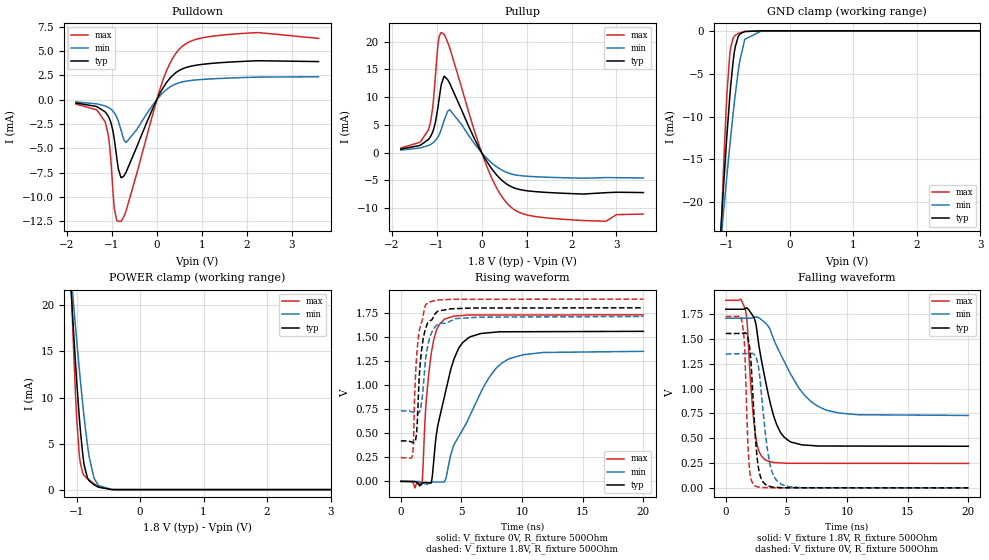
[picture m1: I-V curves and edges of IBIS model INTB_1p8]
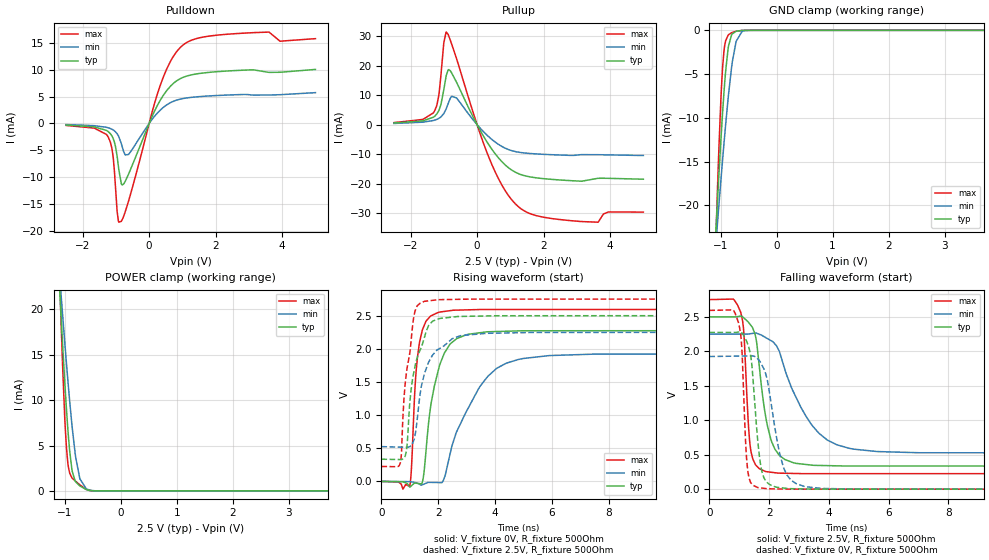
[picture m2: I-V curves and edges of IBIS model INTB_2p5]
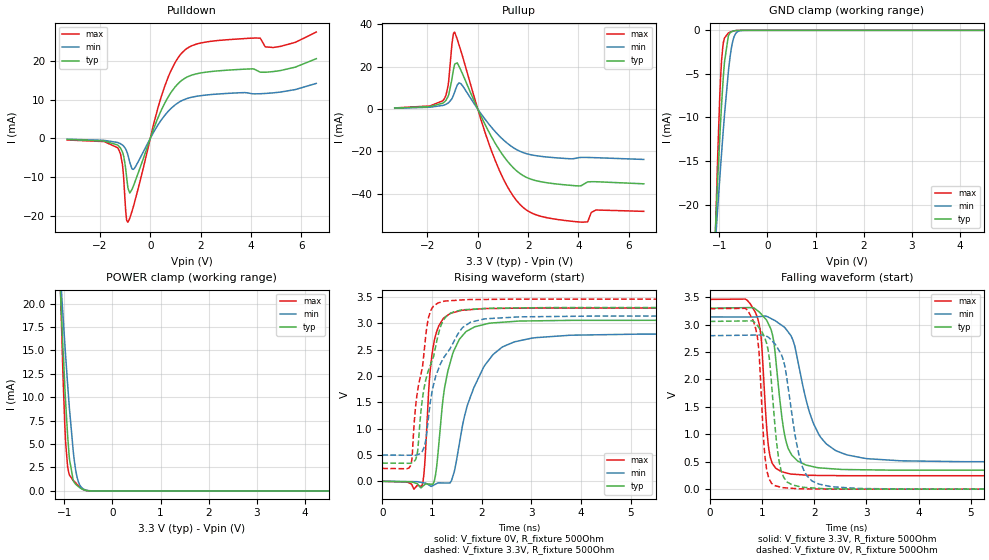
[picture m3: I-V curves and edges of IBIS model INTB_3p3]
|Texas Instruments Incorporated
| Marketing part#   Digital Voltage Range   Package-type   #pins
| LDC1101   1.71V - 3.46V   WSON   10
[IBIS Ver]   4.1
[File name]   ldc1101.ibs
[File Rev]   1.0
[Date]   10/21/2014
[Source]
| Texas Instruments Incorporated.
| 12500 TI Blvd
| Dallas, TX -75243
[Notes]   Revision History:
| Rev 1.0: 10/21/2014
| - Initial version of the model
| - Model generated from simulations in TISPICE
| - C_comp although listed in numerical order of value are
|   obtained from varying PVT conditions. For PVT conditions for
|   each specific value refer the buffer description under
|   respective [Model]. IBIS model user is responsible for using
|   appropriate C_comp to simulate for Signal Integrity.
| - Warnings regarding combined Non-monotonicity of various models have been
|   reviewd and considered minor and can be ignored.
| - Model names with a trailing _1p8 contains the model for
|   1.8V operation. Model names with a trailing _2p5 contains the model
|   for 2.5V operation.Model names with a trailing _3p3 contains the model
|   for 3.3V operation.
[Disclaimer]
| This model is designed as an aid for customers of Texas Instruments.
| TI and its licensors and suppliers make no warranties, either expressed
| or implied, with respect to this  model, including the warranties of
| merchantability or fitness for a particular purpose. The model is
| provided solely on an "as is" basis. The entire risk as to its quality
| and performance is with the customer.
[Copyright]
 (C) Copyright 2014 Texas Instruments Incorporated.All rights reserved.
|   Device
[Component] LDC1101
[Manufacturer]   TI
[Package]  |QFN   64
|   typ   min   max
R_pkg   0.067   0.027   0.083
L_pkg   0.937nH   0.593nH   1.143nH
C_pkg   0.144pF   0.126pF   0.200pF
[Pin]  signal_name   model_name   R_pin   L_pin   C_pin
1   SDO/INTB   INTB   0.07225   0.9423nF   0.10569pF
2   CLKIN   INPUT   0.06963   0.90122nF   0.11966pF
3   SCLK   INPUT   0.06783   0.8751nF   0.1181pF
4   SDI   INPUT   0.06766   0.87334nF   0.11843pF
5   CSB   INPUT   0.07162   0.93329nF   0.10577pF
6   INB   NC   0.03667   0.6676nF   0.1339pF
7   INA   NC   0.03767   0.69067nF   0.16038pF
8   GND   GND   0.03452   0.60581nF   0.15824pF
9   VDD   POWER   0.0342   0.59712nF   0.15278pF
10   CLDO   NC   0.0717   0.92726nF   0.10658pF
|   Model Selectors
[Model Selector]  INTB
INTB_1p8  output buffer at 1.8V operation.
INTB_2p5  output buffer at 2.5V operation.
INTB_3p3  output buffer at 3.3V operation.
[Model Selector]  INPUT
SCLK_1p8  output buffer at 1.8V operation.
SCLK_2p5  output buffer at 2.5V operation.
SCLK_3p3  output buffer at 3.3V operation.
| Models and submodels in the file (6): INTB_1p8 (I/O), INTB_2p5 (I/O), INTB_3p3 (I/O), SCLK_1p8 (Input), SCLK_2p5 (Input), SCLK_3p3 (Input)
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|   Model
[Model]   INTB_1p8
Model_type   I/O
Polarity   Non-Inverting
Enable   Active-Low
Vinl = 0.54
Vinh = 1.26
Vmeas = 0.9
Vref = 0
Cref = 1pF
Rref = 100000
|   typ   min   max
C_comp   0.827pF   0.793pF   0.868pF
[Voltage Range]   1.8   1.71   1.89
[Temperature Range]   27   125   -40
[Pullup Reference]   1.8   1.71   1.89
[Pulldown Reference]   0   0   0
[Power Clamp Reference]   1.8   1.71   1.89
[GND Clamp Reference]   0   0   0
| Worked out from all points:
|   slope of the pulldown table from 0 to 0.27 V, typ, clamps not added: 130 ohm
|   slope of the pullup table from 0 to 0.27 V, typ, clamps not added: 80 ohm
|   GND clamp passes 1 mA (typ) near -0.83 V on its own axis
|   POWER clamp passes 1 mA (typ) near -0.80 V on its own axis
|   falling waveform, V_fixture 1.8V, R_fixture 500Ohm: 20-80 % time 1.4ns typ, 2.66ns min, 587ps max; typ from 1.8 V to 0.419 V
|   rising waveform, V_fixture 0V, R_fixture 500Ohm: 20-80 % time 1.54ns typ, 3.19ns min, 692ps max; typ from 0 V to 1.56 V
|   rising waveform, V_fixture 1.8V, R_fixture 500Ohm: 20-80 % time 531ps typ, 637ps min, 447ps max; typ from 0.419 V to 1.8 V
|   falling waveform, V_fixture 0V, R_fixture 500Ohm: 20-80 % time 493ps typ, 755ps min, 297ps max; typ from 1.56 V to 0 V
[Pulldown]
|   Voltage   I(typ)   I(min)   I(max)
-1.8V     -336.3uA   -230.4uA   -447.7uA
-1.357V   -678.6uA   -412.5uA   -1.012mA
-1.152V   -1.24mA    -641.7uA   -2.261mA
-1.049V   -2.004mA   -876.5uA   -4.803mA
-946.8mV  -4.023mA   -1.336mA   -11.16mA
-892.8mV  -5.91mA    -1.773mA   -12.37mA
-801mV    -7.966mA   -3.049mA   -12.48mA
-682.2mV  -7.425mA   -4.392mA   -11.39mA
117mV     1.045mA    623.4uA    1.749mA
538.2mV   3.104mA    1.8mA      5.371mA
1.899V    3.933mA    2.274mA    6.804mA
3.6V      3.919mA    2.358mA    6.302mA
[GND Clamp]
|   Voltage   I(typ)   I(min)   I(max)
-1.8V     -120.6mA   -88.57mA   -196.3mA
-1.093V   -24.03mA   -25.16mA   -25.67mA
-1.055V   -19.45mA   -22.03mA   -18.1mA
-995.4mV  -12.68mA   -17.26mA   -8.035mA
-946.8mV  -7.79mA    -13.52mA   -2.868mA
-930.6mV  -6.358mA   -12.32mA   -1.935mA
-876.6mV  -2.636mA   -8.545mA   -652.2uA
-811.8mV  -641.6uA   -4.675mA   -304.6uA
-784.8mV  -359uA     -3.37mA    -230.3uA
-709.2mV  -81.9uA    -992uA     -81.84uA
-444.6mV  -100.8nA   -2.623uA   -20.3nA
3.6V      0A         0A         0A
[Pullup]
|   Voltage   I(typ)   I(min)   I(max)
-1.8V     652.3uA    478.7uA    841.9uA
-1.384V   1.299mA    843.4uA    1.858mA
-1.184V   2.391mA    1.309mA    4.139mA
-1.093V   3.712mA    1.732mA    8.059mA
-973.8mV  8.197mA    2.83mA     19.49mA
-898.2mV  12.34mA    4.232mA    21.64mA
-833.4mV  13.78mA    5.911mA    21.28mA
-709.2mV  12.44mA    7.72mA     18.83mA
68.4mV    -966.5uA   -617uA     -1.527mA
613.8mV   -5.931mA   -3.713mA   -9.529mA
1.975V    -7.359mA   -4.541mA   -12.08mA
3.6V      -7.18mA    -4.556mA   -11.05mA
[POWER Clamp]
|   Voltage   I(typ)   I(min)   I(max)
-1.8V     116.8mA    87.13mA    188mA
-1.093V   22.48mA    23.87mA    23.88mA
-1.06V    18.67mA    21.21mA    17.71mA
-1.001V   12.14mA    16.47mA    8.209mA
-946.8mV  7.028mA    12.4mA     3.206mA
-903.6mV  3.914mA    9.363mA    1.825mA
-876.6mV  2.568mA    7.609mA    1.493mA
-801mV    957uA      3.559mA    1.042mA
-725.4mV  531.3uA    1.252mA    646.1uA
-655.2mV  264.8uA    440.2uA    306.4uA
-444.6mV  3.686uA    12.87uA    1.63uA
3.6V      0A         0A         0A
[Ramp]
R_load = 500
|   typ   min   max
dV/dt_r   0.933471/1.5386e-09   0.809123/3.18535e-09   1.03613/6.85503e-10
dV/dt_f   0.828579/1.39636e-09   0.588178/2.65405e-09   0.9861/5.85084e-10
[Falling Waveform]
V_fixture = 1.8V
V_fixture_min = 1.71V
V_fixture_max = 1.89V
R_fixture = 500Ohm
C_fixture = 0F
|   Time   V(typ)   V(min)   V(max)
0s        1.8V       1.71V      1.89V
1.219ns   1.799V     1.71V      1.902V
1.63ns    1.808V     1.71V      1.788V
2.415ns   1.686V     1.72V      562.5mV
3.241ns   1.099V     1.664V     283.3mV
3.994ns   708.3mV    1.484V     255.4mV
4.823ns   509.5mV    1.273V     249.3mV
6.519ns   431.2mV    930.5mV    247.5mV
8.115ns   421.7mV    792mV      247.4mV
20ns      419mV      729.7mV    246.5mV
[Rising Waveform]
V_fixture = 0V
V_fixture_min = 0V
V_fixture_max = 0V
R_fixture = 500Ohm
C_fixture = 0F
|   Time   V(typ)   V(min)   V(max)
0s        3.042nV    52.01nV    1.465nV
1.72ns    -21.89mV   -11.15mV   -32.73mV
2.079ns   -12.56mV   -28.1mV    808.2mV
2.481ns   -16.96mV   -12.94mV   1.302V
2.927ns   483.4mV    -6.927mV   1.564V
3.566ns   863.7mV    -7.019mV   1.678V
4.336ns   1.249V     367.4mV    1.713V
5.108ns   1.44V      539mV      1.721V
8.246ns   1.551V     1.219V     1.725V
20ns      1.556V     1.349V     1.727V
[Rising Waveform]
V_fixture = 1.8V
V_fixture_min = 1.71V
V_fixture_max = 1.89V
R_fixture = 500Ohm
C_fixture = 0F
|   Time   V(typ)   V(min)   V(max)
0s        419mV      729.7mV    246.5mV
959.8ps   405.7mV    717.9mV    272.1mV
1.041ns   402.7mV    714.2mV    410.8mV
1.213ns   426.2mV    706.5mV    1.108V
1.395ns   723.9mV    702.1mV    1.436V
1.685ns   1.338V     797.6mV    1.639V
2.207ns   1.643V     1.399V     1.854V
2.906ns   1.749V     1.615V     1.879V
4.522ns   1.791V     1.688V     1.889V
20ns      1.8V       1.71V      1.89V
[Falling Waveform]
|Gnd
V_fixture = 0V
V_fixture_min = 0V
V_fixture_max = 0V
R_fixture = 500Ohm
C_fixture = 0F
|   Time   V(typ)   V(min)   V(max)
0s        1.556V     1.349V     1.727V
1.354ns   1.557V     1.352V     1.663V
1.56ns    1.562V     1.353V     1.409V
1.795ns   1.524V     1.353V     546mV
1.927ns   1.446V     1.354V     229.4mV
2.415ns   563.4mV    1.332V     19.53mV
2.764ns   154.3mV    1.161V     6.042mV
3.607ns   15.45mV    260.5mV    487.1uV
4.559ns   2.439mV    37.84mV    407.4uV
20ns      13.76nV    93.77nV    4.829nV
|   Model
[Model]   INTB_2p5
Model_type   I/O
Polarity   Non-Inverting
Enable   Active-Low
Vinl = 0.75
Vinh = 1.75
Vmeas = 1.25
Vref = 0
Cref = 1pF
Rref = 100000
|   typ   min   max
C_comp   0.827pF   0.793pF   0.868pF
[Voltage Range]   2.5   2.25   2.75
[Temperature Range]   27   125   -40
[Pullup Reference]   2.5   2.25   2.75
[Pulldown Reference]   0   0   -0
[Power Clamp Reference]   2.5   2.25   2.75
[GND Clamp Reference]   0   0   0
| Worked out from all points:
|   slope of the pulldown table from 0 to 0.375 V, typ, clamps not added: 79 ohm
|   slope of the pullup table from 0 to 0.375 V, typ, clamps not added: 52.1 ohm
|   GND clamp passes 1 mA (typ) near -0.82 V on its own axis
|   POWER clamp passes 1 mA (typ) near -0.81 V on its own axis
|   falling waveform, V_fixture 2.5V, R_fixture 500Ohm: 20-80 % time 432ps typ, 1.14ns min, 184ps max; typ from 2.5 V to 0.334 V
|   rising waveform, V_fixture 0V, R_fixture 500Ohm: 20-80 % time 539ps typ, 1.26ns min, 242ps max; typ from 0 V to 2.27 V
|   rising waveform, V_fixture 2.5V, R_fixture 500Ohm: 20-80 % time 503ps typ, 561ps min, 339ps max; typ from 0.334 V to 2.5 V
|   falling waveform, V_fixture 0V, R_fixture 500Ohm: 20-80 % time 263ps typ, 478ps min, 153ps max; typ from 2.27 V to 0 V
[Pulldown]
|   Voltage   I(typ)   I(min)   I(max)
-2.5V     -286uA     -200.7uA   -364.7uA
-1.653V   -630.8uA   -404.1uA   -862uA
-1.225V   -1.546mA   -811.9uA   -2.588mA
-1.09V    -2.686mA   -1.17mA    -5.892mA
-962.5mV  -6.113mA   -1.915mA   -16.44mA
-910mV    -8.699mA   -2.493mA   -18.41mA
-812.5mV  -11.47mA   -4.284mA   -17.99mA
-617.5mV  -9.426mA   -5.786mA   -14.45mA
327.5mV   4.261mA    2.451mA    6.995mA
957.5mV   8.425mA    4.574mA    14.31mA
2.728V    9.913mA    5.387mA    16.81mA
5V        10.08mA    5.752mA    15.83mA
[GND Clamp]
|   Voltage   I(typ)   I(min)   I(max)
-2.5V     -220.6mA   -154mA     -373.8mA
-1.143V   -30.31mA   -29.38mA   -36.4mA
-1.067V   -20.97mA   -23.08mA   -20.57mA
-1.052V   -19.17mA   -21.85mA   -17.66mA
-992.5mV  -12.37mA   -17.03mA   -7.632mA
-962.5mV  -9.283mA   -14.71mA   -4.145mA
-940mV    -7.174mA   -13.01mA   -2.432mA
-865mV    -2.088mA   -7.79mA    -553uA
-805mV    -551.9uA   -4.326mA   -284.3uA
-722.5mV  -106.5uA   -1.271mA   -101.6uA
-550mV    -2.125uA   -30.09uA   -1.294uA
5V        0A         0A         0A
[Pullup]
|   Voltage   I(typ)   I(min)   I(max)
-2.5V     535.2uA    389.6uA    684.5uA
-1.285V   2.751mA    1.489mA    4.495mA
-1.15V    4.763mA    2.122mA    9.98mA
-1V       11.85mA    3.753mA    27.79mA
-925mV    16.73mA    5.437mA    31.41mA
-850mV    18.68mA    7.715mA    30.06mA
-617.5mV  14.39mA    9.063mA    22.43mA
327.5mV   -6.394mA   -3.871mA   -10.33mA
1.167V    -16.24mA   -9.188mA   -27.08mA
1.798V    -18.08mA   -9.952mA   -30.93mA
3.147V    -19.2mA    -10.19mA   -32.9mA
5V        -18.52mA   -10.48mA   -29.68mA
[POWER Clamp]
|   Voltage   I(typ)   I(min)   I(max)
-2.5V     214.8mA    152.6mA    359mA
-1.15V    29.5mA     28.69mA    35.7mA
-1.075V   20.4mA     22.42mA    20.47mA
-1.067V   19.52mA    21.81mA    19.06mA
-1V       12.05mA    16.41mA    8.104mA
-970mV    9.092mA    14.12mA    4.83mA
-940mV    6.469mA    11.9mA     2.87mA
-872.5mV  2.406mA    7.354mA    1.458mA
-805mV    992.7uA    3.733mA    1.062mA
-730mV    551.7uA    1.342mA    671.2uA
-617.5mV  161.2uA    254.8uA    175.1uA
5V        0A         0A         0A
[Ramp]
R_load = 500
|   typ   min   max
dV/dt_r   1.36448/5.34294e-10   1.15475/1.25777e-09   1.55607/2.4163e-10
dV/dt_f   1.29952/4.27066e-10   1.0354/1.13003e-09   1.51514/1.83827e-10
[Falling Waveform]
V_fixture = 2.5V
V_fixture_min = 2.25V
V_fixture_max = 2.75V
R_fixture = 500Ohm
C_fixture = 0F
|   Time   V(typ)   V(min)   V(max)
0s        2.5V       2.25V      2.75V
1.042ns   2.512V     2.249V     2.574V
1.158ns   2.483V     2.249V     2.244V
1.385ns   2.379V     2.256V     567.8mV
1.583ns   2.128V     2.262V     336.1mV
1.862ns   1.11V      2.205V     259.5mV
2.521ns   431.3mV    1.743V     230.8mV
3.459ns   347.2mV    913.6mV    225.4mV
4.681ns   335.5mV    592.7mV    225.4mV
20ns      334.1mV    524.3mV    224.8mV
[Rising Waveform]
V_fixture = 0V
V_fixture_min = 0V
V_fixture_max = 0V
R_fixture = 500Ohm
C_fixture = 0F
|   Time   V(typ)   V(min)   V(max)
0s        2.164nV    45.82nV    1.193nV
995.4ps   -84.78mV   -3.588mV   -62.6mV
1.202ns   -26.46mV   -18.48mV   1.549V
1.334ns   -33.31mV   -42.21mV   2.076V
1.473ns   52.44mV    -45.51mV   2.317V
1.741ns   1.154V     -14.99mV   2.496V
1.988ns   1.65V      -17.49mV   2.547V
3.459ns   2.241V     1.423V     2.592V
4.833ns   2.27V      1.84V      2.592V
20ns      2.274V     1.925V     2.593V
[Rising Waveform]
V_fixture = 2.5V
V_fixture_min = 2.25V
V_fixture_max = 2.75V
R_fixture = 500Ohm
C_fixture = 0F
|   Time   V(typ)   V(min)   V(max)
0s        334.1mV    524.3mV    224.8mV
663.6ps   329.5mV    516.6mV    275.6mV
876.9ps   451.6mV    514.1mV    1.626V
1.004ns   1.212V     524.2mV    1.954V
1.13ns    1.623V     609.1mV    2.459V
1.507ns   2.162V     1.611V     2.715V
1.807ns   2.419V     1.907V     2.731V
2.492ns   2.478V     2.152V     2.744V
3.705ns   2.495V     2.233V     2.749V
20ns      2.5V       2.25V      2.75V
[Falling Waveform]
|Gnd
V_fixture = 0V
V_fixture_min = 0V
V_fixture_max = 0V
R_fixture = 500Ohm
C_fixture = 0F
|   Time   V(typ)   V(min)   V(max)
0s        2.274V     1.925V     2.593V
972.3ps   2.28V      1.93V      2.417V
1.087ns   2.268V     1.931V     2.039V
1.276ns   2.113V     1.932V     298.4mV
1.417ns   1.822V     1.933V     78.44mV
1.607ns   763.7mV    1.897V     25.95mV
1.819ns   171.4mV    1.75V      12.86mV
2.492ns   15.68mV    303.6mV    1.677mV
3.165ns   3.772mV    41.04mV    385.7uV
20ns      6.394nV    60.83nV    2.527nV
|   Model
[Model]   INTB_3p3
Model_type   I/O
Polarity   Non-Inverting
Enable   Active-Low
Vinl = 0.99
Vinh = 2.31
Vmeas = 1.65
Vref = 0
Cref = 1pF
Rref = 100000
|   typ   min   max
C_comp   0.827pF   0.793pF   0.868pF
[Voltage Range]   3.3   3.14   3.46
[Temperature Range]   27   125   -40
[Pullup Reference]   3.3   3.14   3.46
[Pulldown Reference]   0   0   0
[Power Clamp Reference]   3.3   3.14   3.46
[GND Clamp Reference]   0   0   0
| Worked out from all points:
|   slope of the pulldown table from 0 to 0.495 V, typ, clamps not added: 61.8 ohm
|   slope of the pullup table from 0 to 0.495 V, typ, clamps not added: 41.4 ohm
|   GND clamp passes 1 mA (typ) near -0.82 V on its own axis
|   POWER clamp passes 1 mA (typ) near -0.81 V on its own axis
|   falling waveform, V_fixture 3.3V, R_fixture 500Ohm: 20-80 % time 223ps typ, 447ps min, 136ps max; typ from 3.3 V to 0.346 V
|   rising waveform, V_fixture 0V, R_fixture 500Ohm: 20-80 % time 297ps typ, 569ps min, 164ps max; typ from 0 V to 3.06 V
|   rising waveform, V_fixture 3.3V, R_fixture 500Ohm: 20-80 % time 364ps typ, 509ps min, 254ps max; typ from 0.346 V to 3.3 V
|   falling waveform, V_fixture 0V, R_fixture 500Ohm: 20-80 % time 181ps typ, 289ps min, 122ps max; typ from 3.06 V to 0 V
[Pulldown]
|   Voltage   I(typ)   I(min)   I(max)
-3.3V     -247.8uA   -199.8uA   -395.2uA
-1.29V    -1.724mA   -1.053mA   -2.459mA
-1.102V   -3.533mA   -1.699mA   -6.822mA
-973.5mV  -7.984mA   -2.771mA   -18.83mA
-894.3mV  -12.38mA   -4.103mA   -21.53mA
-815.1mV  -14.05mA   -6.096mA   -20.54mA
-636.9mV  -11.66mA   -7.736mA   -16.72mA
432.3mV   7.171mA    4.689mA    10.63mA
1.264V    14.98mA    9.747mA    22.03mA
3.897V    17.85mA    11.68mA    25.74mA
5.174V    17.45mA    11.92mA    23.66mA
6.6V      20.5mA     14.15mA    27.34mA
[GND Clamp]
|   Voltage   I(typ)   I(min)   I(max)
-3.3V     -336.1mA   -229.7mA   -578mA
-1.082V   -22.78mA   -24.31mA   -23.57mA
-1.073V   -21.57mA   -23.49mA   -21.57mA
-1.043V   -18.03mA   -21.05mA   -15.85mA
-993.3mV  -12.45mA   -17.09mA   -7.742mA
-953.7mV  -8.434mA   -14.04mA   -3.382mA
-894.3mV  -3.652mA   -9.739mA   -877.6uA
-815.1mV  -690.8uA   -4.848mA   -315.1uA
-765.6mV  -244.4uA   -2.582mA   -184.9uA
-676.5mV  -41.86uA   -513.7uA   -44.42uA
-518.1mV  -896.7nA   -14.44uA   -415.7nA
6.6V      0A         0A         0A
[Pullup]
|   Voltage   I(typ)   I(min)   I(max)
-3.3V     449.8uA    359.3uA    530.3uA
-1.36V    3.018mA    1.808mA    4.322mA
-1.181V   5.896mA    2.797mA    10.87mA
-1.023V   14.5mA     4.996mA    30.9mA
-924mV    20.8mA     7.827mA    36.28mA
-676.5mV  18.44mA    12.01mA    27.64mA
570.9mV   -13.6mA    -8.959mA   -20.48mA
1.68V     -30.4mA    -19.91mA   -44.99mA
2.472V    -34.16mA   -22.23mA   -50.43mA
4.155V    -35.82mA   -22.8mA    -53.33mA
4.699V    -34.25mA   -22.93mA   -47.57mA
6.6V      -35.24mA   -23.75mA   -48.22mA
[POWER Clamp]
|   Voltage   I(typ)   I(min)   I(max)
-3.3V     327.9mA    228.3mA    556.1mA
-1.082V   21.27mA    23.03mA    21.89mA
-1.073V   20.1mA     22.21mA    20mA
-1.033V   15.58mA    19.01mA    12.97mA
-993.3mV  11.37mA    15.89mA    7.264mA
-973.5mV  9.423mA    14.38mA    5.144mA
-933.9mV  5.988mA    11.47mA    2.615mA
-894.3mV  3.395mA    8.745mA    1.686mA
-775.5mV  778.9uA    2.571mA    916.2uA
-706.2mV  450uA      938.3uA    543.9uA
-607.2mV  138.2uA    219.3uA    146.6uA
6.6V      0A         0A         0A
[Ramp]
R_load = 500
|   typ   min   max
dV/dt_r   1.83494/2.96967e-10   1.67884/5.65806e-10   1.97447/1.63282e-10
dV/dt_f   1.77259/2.22622e-10   1.58479/4.43538e-10   1.92932/1.34037e-10
[Falling Waveform]
V_fixture = 3.3V
V_fixture_min = 3.14V
V_fixture_max = 3.46V
R_fixture = 500Ohm
C_fixture = 0F
|   Time   V(typ)   V(min)   V(max)
0s        3.3V       3.14V      3.46V
876.6ps   3.282V     3.139V     3.217V
984.2ps   3.193V     3.149V     2.754V
1.093ns   3.075V     3.148V     1.089V
1.197ns   2.829V     3.099V     470.7mV
1.41ns    1.122V     2.966V     310.8mV
1.527ns   698.4mV    2.834V     280.3mV
2.089ns   389.7mV    997.6mV    250.5mV
2.949ns   353.3mV    564.7mV    244.9mV
20ns      345.7mV    498.7mV    244.5mV
[Rising Waveform]
V_fixture = 0V
V_fixture_min = 0V
V_fixture_max = 0V
R_fixture = 500Ohm
C_fixture = 0F
|   Time   V(typ)   V(min)   V(max)
0s        2.131nV    59.1nV     1.251nV
801.4ps   -105.8mV   -23.6mV    -75.41mV
960ps     -52.79mV   -82.97mV   2.055V
1.026ns   -48.66mV   -77.67mV   2.56V
1.254ns   1.776V     -31.64mV   3.111V
1.393ns   2.338V     11.19mV    3.193V
1.578ns   2.725V     857.6mV    3.242V
2.071ns   2.982V     2.211V     3.279V
3.095ns   3.047V     2.728V     3.29V
20ns      3.058V     2.798V     3.291V
[Rising Waveform]
V_fixture = 3.3V
V_fixture_min = 3.14V
V_fixture_max = 3.46V
R_fixture = 500Ohm
C_fixture = 0F
|   Time   V(typ)   V(min)   V(max)
0s        345.7mV    498.7mV    244.5mV
570.4ps   342.3mV    495mV      298.6mV
674.9ps   421.2mV    496.6mV    1.452V
847.4ps   1.8V       657.4mV    2.508V
932.6ps   2.111V     1.229V     3.116V
1.079ns   2.581V     2.006V     3.358V
1.25ns    3.085V     2.365V     3.42V
1.777ns   3.265V     3.02V      3.45V
2.773ns   3.293V     3.122V     3.459V
20ns      3.3V       3.14V      3.46V
[Falling Waveform]
|Gnd
V_fixture = 0V
V_fixture_min = 0V
V_fixture_max = 0V
R_fixture = 500Ohm
C_fixture = 0F
|   Time   V(typ)   V(min)   V(max)
0s        3.058V     2.798V     3.291V
827.5ps   3.062V     2.809V     3.08V
938.6ps   2.949V     2.81V      2.552V
1.016ns   2.838V     2.811V     1.169V
1.132ns   2.441V     2.763V     195.9mV
1.279ns   856.3mV    2.605V     56.47mV
1.377ns   312.5mV    2.441V     30.95mV
1.777ns   35.06mV    401.7mV    5.866mV
2.324ns   7.725mV    46.48mV    1.074mV
20ns      4.696nV    66.66nV    2.215nV
